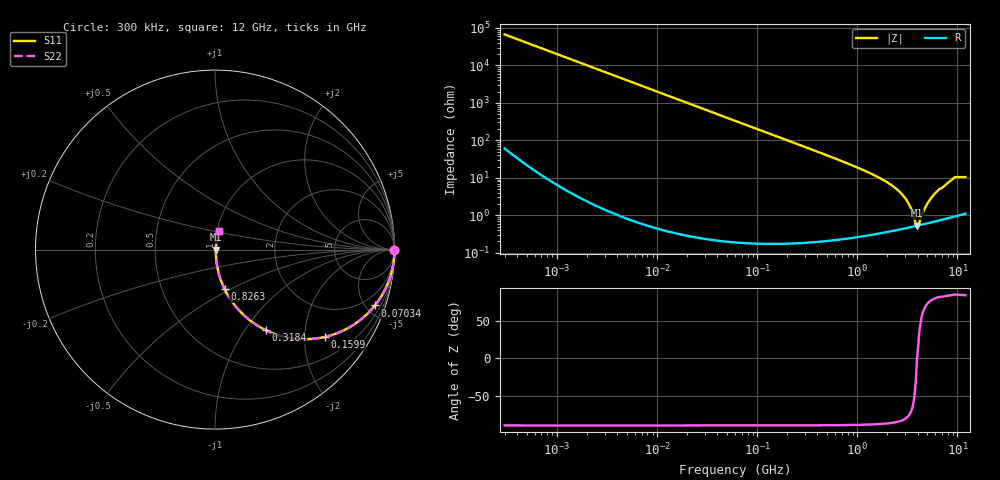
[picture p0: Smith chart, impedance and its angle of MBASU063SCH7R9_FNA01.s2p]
! MBASU063SCH7R9_FNA01  S-PARAMETER MODEL  ( General Type )
! Model Generated by TAIYO YUDEN Corporation (http://www.ty-top.com)
! Version 1.0
! TAIYO YUDEN Control No. 130801
! Copyright(c) 2013 TAIYO YUDEN CO.,LTD. All Rights Reserved.
! Product Description (link to TY-COMPAS)
! https://ds.yuden.co.jp/TYCOMPAS/or/detail?pn=MBASU063SCH7R9DFNA01&u=M
! Products Name : Multilayer Ceramic Capacitors
! Characteristics :
!  Capacitance : 7.9 pF , Rated Voltage : 50V , TCC : CH / C0H
!  Case Size : 0.6 x 0.3 / 0.024 x 0.012 [mm/inch] , Thickness : 0.3 / 0.012 [mm/inch]
!  (Conditions: Temperature = 25 degC , DC Bias Current/Voltage = 0A / 0V)
! External Node Assignments :
!  1  o---| |---o  2
! GND o---------o GND
! Frequency Range : 0.3MHz  -  12000MHz  [ 401 STEP ]
# MHz S RI R 50
! Freq[MHz].  S11 Real  S11 Imag  S21 Real  S21 Imag  S12 Real  S12 Imag  S22 Real  S22 Imag
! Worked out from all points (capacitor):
!   401 points, 300 kHz to 12 GHz, reference 50 ohm
!   read as one part in series: C = 7.91 pF near 316.3 kHz
!   lowest |Z| = 525 mohm at 3.944 GHz (marker M1)
!   series resonance near 3.953 GHz, so ESL is about 200 pH
!   S11 on the Smith chart (normalised r, x): 300 kHz: open; 70.34 MHz: 1.00, -5.72; 159.9 MHz: 1.00, -2.51; 318.4 MHz: 1.00, -1.26; 826.3 MHz: 1.00, -0.47; 12 GHz: 1.02, +0.21
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0.3  1 -0.00149  3.57e-06 0.00149  3.57e-06 0.00149  1 -0.00149
1.769972  0.9999 -0.00879  7.94e-05 0.00879  7.94e-05 0.00879  0.9999 -0.00879
10.44266  0.9973 -0.0517  0.0027 0.0517  0.0027 0.0517  0.9973 -0.0517
27.10171  0.9822 -0.1322  0.0178 0.1322  0.0178 0.1322  0.9822 -0.1322
60  0.9182 -0.2737  0.0818 0.2737  0.0818 0.2737  0.9182 -0.2737
70.33673  0.891 -0.3114  0.109 0.3114  0.109 0.3114  0.891 -0.3114
159.8975  0.6122 -0.4866  0.3878 0.4866  0.3878 0.4866  0.6122 -0.4866
318.4019  0.2835 -0.4492  0.7165 0.4492  0.7165 0.4492  0.2835 -0.4492
353.9943  0.2421 -0.4267  0.7579 0.4267  0.7579 0.4267  0.2421 -0.4267
826.3444  0.0535 -0.22  0.9465 0.22  0.9465 0.22  0.0535 -0.22
1441.349  0.0174 -0.1186  0.9826 0.1186  0.9826 0.1186  0.0174 -0.1186
2088.533  0.00841 -0.0687  0.9916 0.0687  0.9916 0.0687  0.00841 -0.0687
2581.562  0.00606 -0.0443  0.9939 0.0443  0.9939 0.0443  0.00606 -0.0443
3026.31  0.00522 -0.0273  0.9948 0.0273  0.9948 0.0273  0.00522 -0.0273
3364.605  0.00502 -0.0163  0.995 0.0163  0.995 0.0163  0.00502 -0.0163
3740.715  0.00509 -0.00559  0.9949 0.00559  0.9949 0.00559  0.00509 -0.00559
3944.255  0.00522 -0.00013  0.9948 0.00013  0.9948 0.00013  0.00522 -0.00013
4158.869  0.00541 0.00371  0.9946 -0.00371  0.9946 -0.00371  0.00541 0.00371
5006.236  0.00643 0.0194  0.9936 -0.0194  0.9936 -0.0194  0.00643 0.0194
6188.031  0.00868 0.0417  0.9913 -0.0417  0.9913 -0.0417  0.00868 0.0417
9207.246  0.0183 0.0954  0.9817 -0.0954  0.9817 -0.0954  0.0183 0.0954
12000  0.0213 0.101  0.9787 -0.101  0.9787 -0.101  0.0213 0.101
